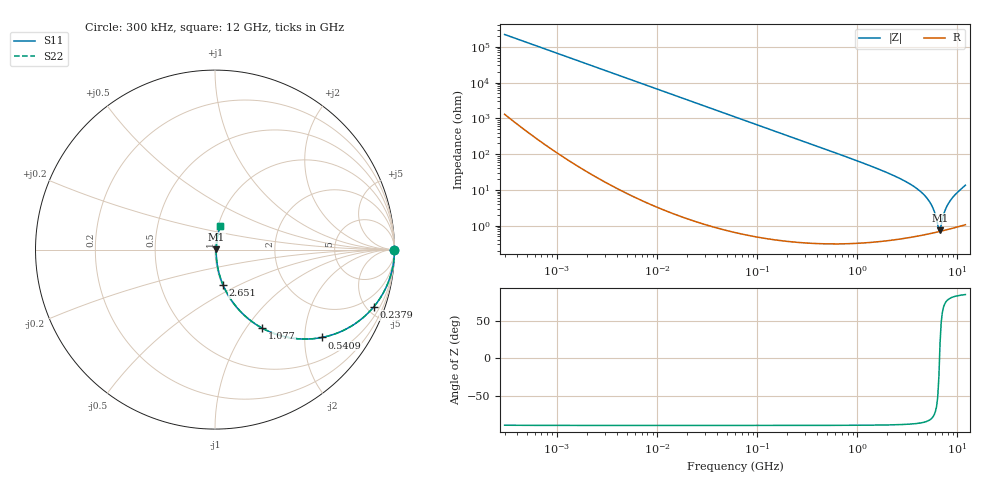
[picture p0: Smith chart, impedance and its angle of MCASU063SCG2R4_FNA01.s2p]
! MCASU063SCG2R4_FNA01  S-PARAMETER MODEL  ( Standard Model )
! Model Generated by TAIYO YUDEN Corporation (http://www.ty-top.com)
! Version 1.0
! TAIYO YUDEN Control No. 230609
! Copyright(c) 2023 TAIYO YUDEN CO.,LTD. All Rights Reserved.
! Product Description (link to TY-COMPAS)
! https://ds.yuden.co.jp/TYCOMPAS/or/detail?pn=MCASU063SCG2R4BFNA01&u=M
! Products Name : Multilayer Ceramic Capacitors
! Characteristics :
!  Capacitance : 2.4 [pF] , Rated Voltage : 50 [V] , TCC : CG / C0G
!  Case Size : 0.6 x 0.3 / 0.024 x 0.012 [mm/inch] , Thickness : 0.3 / 0.012 [mm/inch]
!  (Conditions: Temperature = 25 [degC] , DC Bias Voltage = 0 [V])
! External Node Assignments :
!  1  o---| |---o  2
! GND o---------o GND
! Frequency Range : 0.3MHz  -  12000MHz  [ 401 STEP ]
# MHZ S RI R 50
! Freq[MHz].  S11 Real  S11 Imag  S21 Real  S21 Imag  S12 Real  S12 Imag  S22 Real  S22 Imag
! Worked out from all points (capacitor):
!   401 points, 300 kHz to 12 GHz, reference 50 ohm
!   read as one part in series: C = 2.41 pF near 316.3 kHz
!   lowest |Z| = 740 mohm at 6.7 GHz (marker M1)
!   series resonance near 6.62 GHz, so ESL is about 240 pH
!   S11 on the Smith chart (normalised r, x): 300 kHz: open; 237.9 MHz: 1.01, -5.55; 540.9 MHz: 1.01, -2.43; 1.077 GHz: 1.01, -1.20; 2.651 GHz: 1.01, -0.42; 12 GHz: 1.02, +0.27
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0.3  1 -0.000454  2.87e-06 0.000454  2.87e-06 0.000454  1 -0.000454
1.769972  1 -0.00268  9.97e-06 0.00268  9.97e-06 0.00268  1 -0.00268
10.44266  0.9997 -0.0158  0.000257 0.0158  0.000257 0.0158  0.9997 -0.0158
60  0.9918 -0.09  0.00822 0.09  0.00822 0.09  0.9918 -0.09
136.3989  0.959 -0.1978  0.041 0.1978  0.041 0.1978  0.959 -0.1978
237.9135  0.8849 -0.3186  0.1151 0.3186  0.1151 0.3186  0.8849 -0.3186
353.9943  0.7759 -0.4161  0.2241 0.4161  0.2241 0.4161  0.7759 -0.4161
540.8523  0.5958 -0.4895  0.4042 0.4895  0.4042 0.4895  0.5958 -0.4895
1076.992  0.2645 -0.4383  0.7355 0.4383  0.7355 0.4383  0.2645 -0.4383
2088.533  0.0783 -0.2619  0.9217 0.2619  0.9217 0.2619  0.0783 -0.2619
2650.866  0.0458 -0.1992  0.9542 0.1992  0.9542 0.1992  0.0458 -0.1992
3841.137  0.0177 -0.1118  0.9823 0.1118  0.9823 0.1118  0.0177 -0.1118
4875.354  0.00947 -0.0613  0.9905 0.0613  0.9905 0.0613  0.00947 -0.0613
5565.855  0.00734 -0.0346  0.9927 0.0346  0.9927 0.0346  0.00734 -0.0346
5868.704  0.00691 -0.024  0.9931 0.024  0.9931 0.024  0.00691 -0.024
6354.153  0.00673 -0.00831  0.9933 0.00831  0.9933 0.00831  0.00673 -0.00831
6699.894  0.0069 0.00253  0.9931 -0.00253  0.9931 -0.00253  0.0069 0.00253
6879.757  0.00707 0.00785  0.9929 -0.00785  0.9929 -0.00785  0.00707 0.00785
7648.807  0.00836 0.0287  0.9916 -0.0287  0.9916 -0.0287  0.00836 0.0287
8281.503  0.00993 0.0441  0.9901 -0.0441  0.9901 -0.0441  0.00993 0.0441
9708.23  0.0149 0.0764  0.9851 -0.0764  0.9851 -0.0764  0.0149 0.0764
12000  0.0278 0.1297  0.9722 -0.1297  0.9722 -0.1297  0.0278 0.1297
